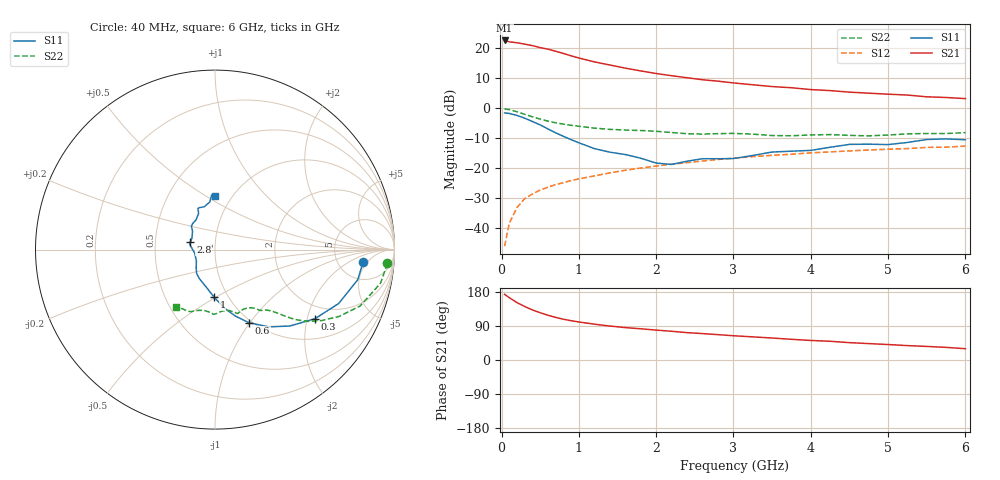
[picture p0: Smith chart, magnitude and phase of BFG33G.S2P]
! Filename:  BFG33G.S2P  Version:  2.0
! Philips part #: BFG 33  Date: Jul 1990
! Bias condition: Vce=5V, Ic=10mA
! IN LINE PINNING: same data as with cross emitter pinning.
#  MHz  S  MA  R  50
! Freq  S11  S21  S12  S22  !GUM [dB]
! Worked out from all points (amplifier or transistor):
!   33 points, 40 MHz to 6 GHz, reference 50 ohm
!   highest |S21| = 22.5 dB at 40 MHz (marker M1)
!   |S21| within 3 dB of that: start of sweep to 614.6 MHz
!   unconditionally stable (mu >= 1): 1.142 GHz to end of sweep
!   at 500 MHz: K = 0.64, MSG = 23.7 dB, |S12| = -27.3 dB
!   at 2.2 GHz: K = 1.20, MAG = 12.0 dB, |S12| = -18.7 dB
!   at 6 GHz: K = 1.36, MAG = 4.3 dB, |S12| = -12.7 dB
!   lowest NFmin = 3.10 dB at 500 MHz
!   S11 on the Smith chart (normalised r, x): 40 MHz: 8.88, -3.92; 300 MHz: 1.57, -2.23; 600 MHz: 0.97, -0.99; 1 GHz: 0.86, -0.49; 2.8 GHz: 0.76, +0.06; 6 GHz: 0.84, +0.55
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40  0.828 -4.8  13.35 173.1  0.005 83.9  0.964 -4.6
100  0.813 -11.9  12.67 164.5  0.012 79.3  0.941 -11.5
200  0.752 -23.5  12.22 151.5  0.022 72.0  0.867 -21.3
300  0.677 -34.7  11.6 141.1  0.031 67.2  0.784 -28.4
400  0.596 -45.6  10.96 132.1  0.037 63.8  0.714 -33.6
500  0.524 -55.2  10.15 124.8  0.043 61.8  0.654 -37.7
600  0.449 -65.1  9.558 118.1  0.048 61.1  0.605 -40.4
700  0.387 -73.0  8.832 112.4  0.053 60.5  0.568 -42.2
800  0.338 -79.6  8.108 107.6  0.057 60.4  0.539 -43.5
900  0.297 -85.3  7.408 103.7  0.062 60.3  0.516 -44.5
1000  0.264 -91.3  6.812 100.3  0.066 60.3  0.496 -45.5
1200  0.211 -104.4  5.875 94.6  0.074 60.2  0.463 -47.5
1400  0.184 -118.2  5.207 89.7  0.083 60.0  0.441 -49.7
1600  0.168 -127.5  4.62 85.5  0.092 59.9  0.43 -52.0
2000  0.121 -149.0  3.756 78.9  0.108 59.4  0.41 -54.5
2200  0.115 -169.8  3.454 75.8  0.116 58.7  0.391 -56.4
2600  0.143 168.9  2.955 69.7  0.131 57.1  0.368 -64.9
2800  0.143 162.9  2.801 66.9  0.139 56.1  0.374 -68.7
3250  0.162 140.6  2.439 61.0  0.155 54.8  0.367 -72.5
4250  0.222 114.3  1.951 49.4  0.186 50.5  0.361 -91.1
5250  0.267 96.2  1.644 38.0  0.211 46.5  0.371 -111.2
6000  0.296 89.6  1.434 29.8  0.232 42.9  0.389 -124.4
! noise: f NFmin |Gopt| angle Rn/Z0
500  3.1  0.528  5.3  1.18
1000  3.1  0.477  12.7  1.33
2000  3.6  0.418  39.1  0.98
